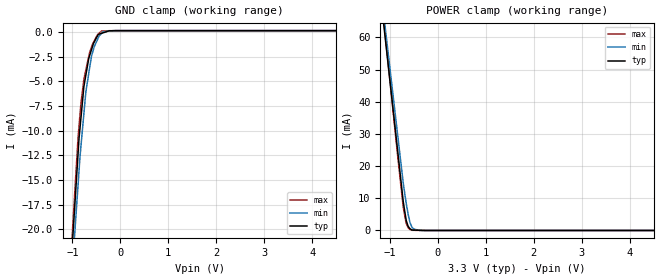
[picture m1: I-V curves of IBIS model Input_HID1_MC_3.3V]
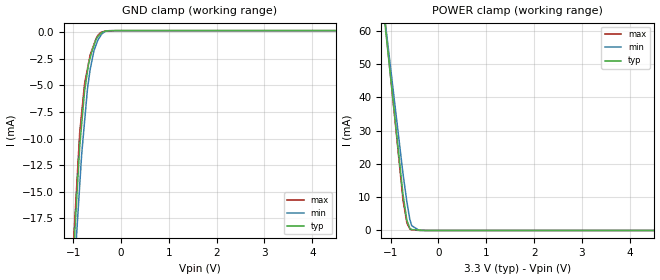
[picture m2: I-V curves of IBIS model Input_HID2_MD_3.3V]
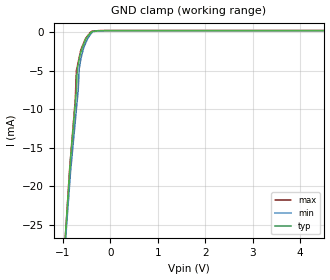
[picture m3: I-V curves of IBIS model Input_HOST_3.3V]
|Texas Instruments Incorporated
|Stereo Audio DAC w/ USB interface,
|Single-Ended Headphone Output and S/PDIF Output
| Marketing part#   Package-type   #pins/pkg drawing
|   PCM2706C   QFP   32
[IBIS Ver]   4.0
[Comment Char] |_char
[File Name]   pcm2706c.ibs
[File Rev]   3.0
[Source]   Texas Instruments Incorporated.
   Analog-eLab, HPA
   12500 TI Blvd
   Dallas, TX -75243
[Date]   10-18-2004
[Notes]   Quality Check of this IBIS model: Model Passes IBIS Check
   Model parses into ICX IS. Simulation done with Hyperlynx.
   1. MIN TYP MAX information is based on Temprature and Voltage
   characteristics only.
[Disclaimer]
| This model is designed as an aid for customers of Texas Instruments.
| TI and its licensors and suppliers make no warranties, either expressed
| or implied, with respect to this  model, including the warranties of
| merchantability or fitness for a particular purpose.
| The model is provided solely on an "as is" basis. The entire risk as to
| its quality and performance is with the customer.
[Copyright]
| (C) Copyright 2011 Texas Instruments Incorporated. All rights reserved.
[Component] PCM2706C
[Manufacturer] TI
[Package]
| variable   typ   min   max
R_pkg  1.8006E-02  1.8006E-02  1.8006E-02
L_pkg  2.1607E-09  2.1607E-09  2.1607E-09
C_pkg  6.0021E-13  6.0021E-13  6.0021E-13
[Pin] signal_name  model_name  R_pin  L_pin C_pin
1   PGND   GND   0.16662   3.74266nF   0.43153pF
2   VCCP   POWER   0.14947   3.32982nF   0.43568pF
3   HOST   Input_HOST_3.3V   0.142   3.08462nF   0.41589pF
4   FUNC3   Input_HID0_MS_3.3V   0.13857   3.02098nF   0.38019pF
5   FUNC0   FUNCX   0.13864   3.02409nF   0.37918pF
6   HID0   Input_HID0_MS_3.3V   0.14117   3.07496nF   0.41438pF
7   HID1   Input_HID1_MC_3.3V   0.14912   3.32922nF   0.43479pF
8   HID2   Input_HID2_MD_3.3V   0.16334   3.69246nF   0.43188pF
9   FSEL   Input_TEST1_3.3V   0.15782   3.60476nF   0.42883pF
10   TEST   Input_TEST0_3.3V   0.13171   3.04522nF   0.42144pF
11   SSPNDB   Output_SSPND_3.3V   0.12033   2.73662nF   0.39319pF
12   XTI   Input_XTI_3.3V   0.12365   2.78238nF   0.36353pF
13   XTO   Output_XTO_3.3V   0.12309   2.77364nF   0.36555pF
14   CK   Output_CK_3.3V   0.12487   2.81072nF   0.39709pF
15   DT   BI_DT_3.3V   0.12313   2.90534nF   0.40917pF
16   PSEL   Input_PSEL_3.3V   0.14419   3.37682nF   0.41439pF
17   DOUT   Output_DOUT_3.3V   0.1537   3.53505nF   0.42278pF
18   FUNC2   FUNCX   0.14215   3.21362nF   0.42852pF
19   FUNC1   FUNCX   0.13732   3.01022nF   0.41183pF
20   DGND   GND   0.13782   3.00898nF   0.3839pF
21   VDD   POWER   0.0749   2.57489nF   0.43767pF
22   D-   USB_3.3V   0.1426   3.09482nF   0.41973pF
23   D+   USB_3.3V   0.15698   3.45354nF   0.44286pF
24   VBUS   POWER   0.15396   3.53072nF   0.41794pF
25   ZGND   GND   0.13421   3.20755nF   0.40592pF
26   AGNDL   GND   0.12267   2.88872nF   0.41489pF
27   VCCL   POWER   0.11998   2.72162nF   0.39703pF
28   VoutL   NC   0.13829   3.01198nF   0.37122pF
29   VoutR   NC   0.13772   3.00294nF   0.37069pF
30   VCCR   POWER   0.12019   2.72542nF   0.39703pF
31   AGNDR   GND   0.12543   2.93375nF   0.41674pF
32   VCOM   POWER   0.13759   3.26032nF   0.40774pF
| Models and submodels in the file (15): Input_HID1_MC_3.3V (Input), Input_HID2_MD_3.3V (Input), Input_HID0_MS_3.3V (Input), Input_HOST_3.3V (Input), Input_PSEL_3.3V (Input), Input_TEST0_3.3V (Input), Input_TEST1_3.3V (Input), Input_XTI_3.3V (Input), Output_CK_3.3V (Output), Output_DOUT_3.3V (Output), FUNCX (I/O), BI_DT_3.3V (I/O), Output_SSPND_3.3V (Output), Output_XTO_3.3V (Output), USB_3.3V (I/O)
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[Model] Input_HID1_MC_3.3V
Model_type Input
Vinl  = 800.000mV
Vinh  = 2.00000V
C_comp  2.00000pF 2.00000pF 2.00000pF
| variable   typ   min   max
[Voltage Range]   3.30000V  3.00000V  3.60000V
[POWER Clamp Reference]  3.30000V  3.00000V  3.60000V
[GND Clamp Reference]   0.00000V  0.00000V  0.00000V
[Temperature Range]   25   85   -25
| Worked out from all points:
|   GND clamp passes 1 mA (typ) near -0.55 V on its own axis
|   POWER clamp passes 1 mA (typ) near -0.60 V on its own axis
[GND Clamp]
-3.3V     -198.8mA   -187mA     -207.8mA
-881.1mV  -12.31mA   -15.49mA   -10.64mA
-861.1mV  -10.77mA   -14.08mA   -9.489mA
-820.8mV  -8.675mA   -11.56mA   -7.169mA
-760.1mV  -5.523mA   -8.271mA   -4.759mA
-719.6mV  -4.376mA   -6.078mA   -3.836mA
-659mV    -2.662mA   -4.201mA   -2.457mA
-603.2mV  -1.796mA   -2.471mA   -1.534mA
-461.8mV  -223.6uA   -588.8uA   -189.1uA
-390.9mV  -110.6uA   -114.1uA   123uA
-110.6mV  144.4uA    171uA      162.2uA
6.6V      144.4uA    171uA      168.5uA
[POWER Clamp]
-3.3V     358.2mA    346.1mA    380.2mA
-1.039V   52.01mA    55.59mA    52.39mA
-842.3mV  25.32mA    30.27mA    23.83mA
-721.1mV  8.907mA    14.7mA     7.145mA
-660.2mV  3.154mA    8.48mA     2.208mA
-619.9mV  1.299mA    5.074mA    839uA
-579.2mV  517uA      2.386mA    287uA
-538.6mV  143.5uA    950.4uA    53uA
-498mV    121.8uA    421.7uA    47.85uA
-381.7mV  59.89uA    0A         33.08uA
6.6V      0A         0A         0A
[Model] Input_HID2_MD_3.3V
Model_type Input
Vinl  = 800.000mV
Vinh  = 2.00000V
C_comp  2.00000pF 2.00000pF 2.00000pF
| variable   typ   min   max
[Voltage Range]   3.30000V  3.00000V  3.60000V
[POWER Clamp Reference]  3.30000V  3.00000V  3.60000V
[GND Clamp Reference]   0.00000V  0.00000V  0.00000V
[Temperature Range]   25   85   -25
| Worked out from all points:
|   GND clamp passes 1 mA (typ) near -0.55 V on its own axis
|   POWER clamp passes 1 mA (typ) near -0.61 V on its own axis
[GND Clamp]
-3.3V     -202.3mA   -188.4mA   -204.3mA
-861.2mV  -10.72mA   -14.36mA   -9.41mA
-820.9mV  -8.663mA   -11.49mA   -7.586mA
-760.1mV  -5.554mA   -8.402mA   -4.835mA
-699.5mV  -3.669mA   -5.325mA   -3.426mA
-643.8mV  -2.39mA    -3.477mA   -2.13mA
-562.3mV  -1.186mA   -1.697mA   -1.114mA
-502mV    -524.1uA   -970uA     -443.3uA
-421mV    -152uA     -289.9uA   1.582uA
-310.9mV  131.6uA    135.8uA    112.4uA
-181.8mV  165.3uA    158.2uA    136.9uA
6.6V      176.1uA    158.9uA    160.8uA
[POWER Clamp]
-3.3V     358.5mA    330.7mA    375.2mA
-1.039V   51.39mA    53.61mA    51.84mA
-741.1mV  10.88mA    17.07mA    9.188mA
-660.1mV  3.071mA    8.621mA    2.296mA
-599.6mV  727.7uA    3.402mA    494.6uA
-559.1mV  265uA      1.442mA    152.2uA
-402.1mV  116.2uA    5.961uA    32.75uA
6.6V      0A         0A         0A
[Model] Input_HOST_3.3V
Model_type Input
Vinl  = 800.000mV
Vinh  = 2.00000V
C_comp  2.00000pF 2.00000pF 2.00000pF
| variable   typ   min   max
[Voltage Range]   3.30000V  3.00000V  3.60000V
[POWER Clamp Reference]  3.30000V  3.00000V  3.60000V
[GND Clamp Reference]   0.00000V  0.00000V  0.00000V
[Temperature Range]   25   85   -25
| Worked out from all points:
|   GND clamp passes 1 mA (typ) near -0.53 V on its own axis
[GND Clamp]
-3.3V     -243.7mA   -224.9mA   -258.1mA
-861.2mV  -18.2mA    -19.8mA    -17.84mA
-840.9mV  -16.33mA   -18.09mA   -16.3mA
-739.7mV  -9.137mA   -11.46mA   -8.638mA
-719.7mV  -7.713mA   -10.15mA   -5.058mA
-699.5mV  -4.792mA   -8.821mA   -4.473mA
-679.1mV  -4.138mA   -7.485mA   -3.884mA
-659mV    -3.493mA   -4.781mA   -3.302mA
-623.6mV  -2.607mA   -3.468mA   -2.28mA
-562.2mV  -1.505mA   -1.988mA   -1.389mA
-380.8mV  64.81uA    5.095uA    131.8uA
6.6V      188.4uA    189.4uA    203.1uA
[POWER Clamp]
| Voltage   I(typ)   I(min)   I(max)
-3.6V     0A         0A         0A
-3.5V     0A         0A         0A
-3.4V     0A         0A         0A
7.2V      0A         0A         0A
